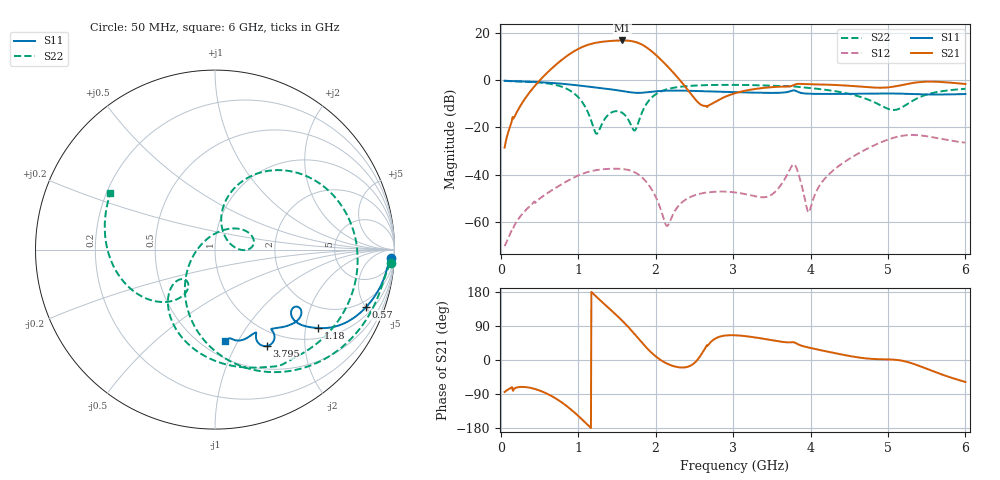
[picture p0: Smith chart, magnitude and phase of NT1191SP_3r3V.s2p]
! Created Wed Apr  6 16:54:32 2022
# hz S ma R 50
! 2 Port Network Data from SP4.SP block
! freq  magS11  angS11  magS21  angS21  magS12  angS12  magS22  angS22
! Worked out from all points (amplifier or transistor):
!   1191 points, 50 MHz to 6 GHz, reference 50 ohm
!   highest |S21| = 16.9 dB at 1.57 GHz (marker M1)
!   |S21| within 3 dB of that: 1.037 GHz to 1.886 GHz (848.2 MHz wide, 58 % of centre)
!   unconditionally stable (mu >= 1): start of sweep to end of sweep
!   at 1.04 GHz: K = 3.54, MAG = 18.5 dB, |S12| = -39.8 dB
!   at 3.025 GHz: K = 55.21, MAG = 0.6 dB, |S12| = -47.5 dB
!   at 6 GHz: K = 4.98, MAG = 2.5 dB, |S12| = -26.4 dB
!   lowest NFmin = 0.54 dB at 850 MHz
!   S11 on the Smith chart (normalised r, x): 50 MHz: 15, -36; 570 MHz: 1.48, -5.04; 1.18 GHz: 1.29, -2.34; 3.795 GHz: 0.79, -1.35; 6 GHz: 0.64, -0.89
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5e7  0.9805 -2.7  0.03753 -84.4  0.0003037 -67.5  0.9812 -4.5
5.7e8  0.9013 -20.7  1.298 -86.3  0.003729 150.9  0.8741 -42.3
7.35e8  0.8623 -26.1  2.304 -104.6  0.005554 133.5  0.7798 -60.8
8.75e8  0.8219 -30.4  3.471 -125.2  0.007566 119.0  0.6334 -81.5
1.045e9  0.7653 -34.7  5.031 -155.9  0.01027 98.7  0.3586 -115.6
1.18e9  0.7204 -37.3  6.009 177.6  0.012 80.8  0.1222 -165.8
1.27e9  0.6924 -38.8  6.435 160.3  0.01274 68.9  0.08651 93.0
1.365e9  0.6633 -40.2  6.729 142.5  0.01318 56.2  0.1693 43.8
1.57e9  0.593 -41.7  7.014 103.4  0.01316 26.2  0.2041 3.6
1.69e9  0.5537 -40.1  6.789 77.3  0.01195 4.3  0.1053 9.2
1.815e9  0.5445 -36.2  5.823 47.8  0.009033 -22.5  0.1915 79.3
1.905e9  0.562 -34.6  4.712 27.6  0.006215 -42.5  0.3581 72.5
2.035e9  0.5908 -35.5  3.096 4.3  0.002518 -74.2  0.5468 53.9
2.15e9  0.6035 -37.7  2.005 -9.8  0.0008154 -160.7  0.649 39.6
2.4e9  0.602 -42.5  0.6769 -18.6  0.003041 111.2  0.7535 16.9
3.025e9  0.5611 -50.9  0.5326 65.3  0.004193 95.7  0.8012 -19.3
3.465e9  0.5422 -54.4  0.7092 53.6  0.003507 139.5  0.774 -41.7
3.795e9  0.6099 -61.7  0.8101 46.1  0.01615 113.0  0.7404 -60.5
3.96e9  0.5221 -63.9  0.8279 33.6  0.001742 109.6  0.6945 -71.3
4.02e9  0.518 -63.6  0.8233 30.8  0.002531 -179.6  0.6795 -75.2
5.01e9  0.5261 -73.3  0.7116 1.6  0.05616 152.4  0.246 -138.1
6e9  0.5122 -83.6  0.8363 -57.9  0.04767 81.0  0.6618 151.7
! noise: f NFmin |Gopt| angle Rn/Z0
5e+07  3.751  0.9699  2.931  27.69
7.1e+08  0.5522  0.7252  20.92  0.3563
1.37e+09  0.6014  0.6482  36.48  0.2782
2.03e+09  0.911  0.5653  50.78  0.2815
2.69e+09  6.163  0.5632  48.89  2.523
3.355e+09  3.005  0.4342  63.44  0.6124
4.015e+09  3.281  0.3809  75.12  0.5636
4.675e+09  4.827  0.3659  74.62  0.9452
5.335e+09  4.528  0.2811  92.66  0.6579
6e+09  4.638  0.204  95.32  0.6456
